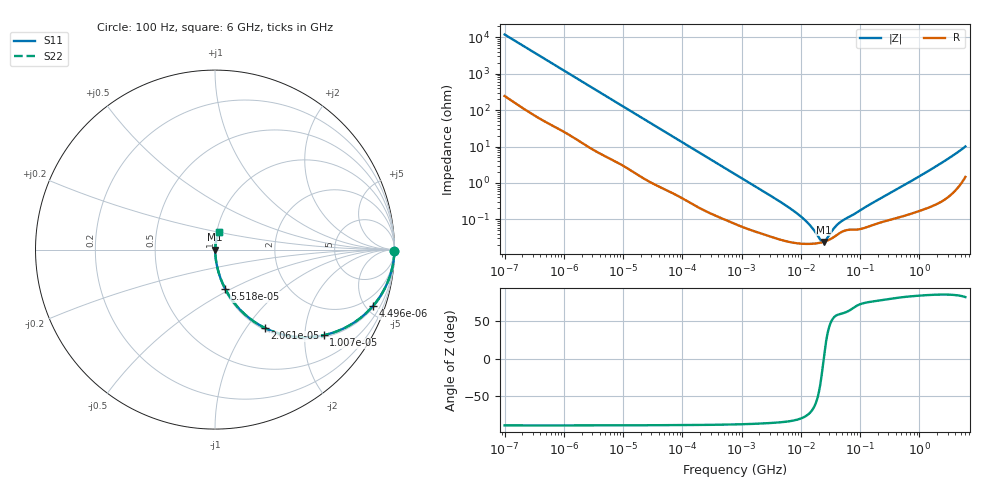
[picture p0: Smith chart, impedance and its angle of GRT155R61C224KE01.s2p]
!Murata Part Number: GRT155R61C224KE01
!These Parameters are Measured in Series Mode Connection
!Data Generated on Jun 19, 2026
!  o--ll--o
!Port1  Port2
!  o------o
!Operation Temp=25[degC], DC Bias Voltage=0[V]
!Freq. Start=100[Hz] Stop=6[GHz] 401[Steps]
# Hz S RI R 50
!Freq.(Hz) S11(Real) S11(Imag) S21(Real) S21(Imag) S12(Real) S12(Imag) S22(Real) S22(Imag)
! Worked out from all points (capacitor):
!   401 points, 100 Hz to 6 GHz, reference 50 ohm
!   read as one part in series: C = 134 nF near 109 Hz
!   lowest |Z| = 24.3 mohm at 24.34 MHz (marker M1)
!   series resonance near 24.38 MHz, so ESL is about 320 pH
!   S11 on the Smith chart (normalised r, x): 100 Hz: open; 4.496 kHz: 1.12, -5.51; 10.07 kHz: 1.06, -2.49; 20.61 kHz: 1.03, -1.23; 55.18 kHz: 1.01, -0.47; 6 GHz: 1.03, +0.20
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100  0.9998 -0.00845  0.000245 0.00845  0.000245 0.00845  0.9998 -0.00845
600  0.9966 -0.0494  0.00342 0.0494  0.00342 0.0494  0.9966 -0.0494
2008  0.9709 -0.1582  0.0291 0.1582  0.0291 0.1582  0.9709 -0.1582
4496  0.8786 -0.3161  0.1214 0.3161  0.1214 0.3161  0.8786 -0.3161
10066  0.6062 -0.4769  0.3938 0.4769  0.3938 0.4769  0.6062 -0.4769
14402  0.4361 -0.4842  0.5639 0.4842  0.5639 0.4842  0.4361 -0.4842
20606  0.2795 -0.4373  0.7205 0.4373  0.7205 0.4373  0.2795 -0.4373
40335  0.0973 -0.2841  0.9027 0.2841  0.9027 0.2841  0.0973 -0.2841
55182  0.0568 -0.2184  0.9432 0.2184  0.9432 0.2184  0.0568 -0.2184
161617  0.00892 -0.0802  0.9911 0.0802  0.9911 0.0802  0.00892 -0.0802
774597  0.00105 -0.0174  0.9989 0.0174  0.9989 0.0174  0.00105 -0.0174
6644369  0.000242 -0.00198  0.9998 0.00198  0.9998 0.00198  0.000242 -0.00198
1.087309e7  0.000216 -0.00105  0.9998 0.00105  0.9998 0.00105  0.000216 -0.00105
1.555665e7  0.000215 -0.000546  0.9998 0.000546  0.9998 0.000546  0.000215 -0.000546
2.128304e7  0.00023 -0.00016  0.9998 0.00016  0.9998 0.00016  0.00023 -0.00016
2.434276e7  0.000243 -1.7e-06  0.9998 1.7e-06  0.9998 1.7e-06  0.000243 -1.7e-06
2.662322e7  0.000254 0.000103  0.9997 -0.000103  0.9997 -0.000103  0.000254 0.000103
3.80911e7  0.000348 0.000522  0.9997 -0.000522  0.9997 -0.000522  0.000348 0.000522
4.764863e7  0.000444 0.00075  0.9996 -0.00075  0.9996 -0.00075  0.000444 0.00075
3.124326e8  0.000989 0.00502  0.999 -0.00502  0.999 -0.00502  0.000989 0.00502
1.791126e9  0.00314 0.0265  0.9969 -0.0265  0.9969 -0.0265  0.00314 0.0265
6e9  0.0238 0.0956  0.9762 -0.0956  0.9762 -0.0956  0.0238 0.0956
